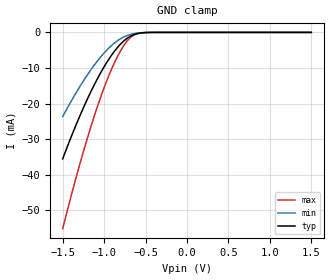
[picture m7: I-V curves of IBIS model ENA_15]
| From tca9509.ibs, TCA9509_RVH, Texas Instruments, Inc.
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[Model]   ENA_15
Model_type  Input
Vinl=0.15
Vinh=1.05
| variable   typ   min   max
C_comp   1.67pF   1.17pF   1.91pF
[Temperature Range]   40   100   -40
| Ambient temperature   25   85   -40
[Voltage range]   1.5   1.35   1.65
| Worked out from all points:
|   GND clamp passes 1 mA (typ) near -0.68 V on its own axis
[GND Clamp]
| ENA_15
|   Voltage   I(typ)   I(min)   I(max)
-1.5V     -35.53mA   -23.65mA   -55.14mA
-1.375V   -28.05mA   -18.4mA    -43.93mA
-1.255V   -21.44mA   -13.8mA    -33.88mA
-1.14V    -15.7mA    -9.862mA   -25.02mA
-1.035V   -11.06mA   -6.72mA    -17.75mA
-935mV    -7.237mA   -4.213mA   -11.67mA
-840mV    -4.263mA   -2.36mA    -6.822mA
-750mV    -2.153mA   -1.149mA   -3.25mA
-670mV    -934.3uA   -505.3uA   -1.19mA
-595mV    -324.9uA   -196.1uA   -314.7uA
-480mV    -38.67uA   -33.04uA   -22.02uA
1.5V      175.6pA    965.7pA    24.92pA
